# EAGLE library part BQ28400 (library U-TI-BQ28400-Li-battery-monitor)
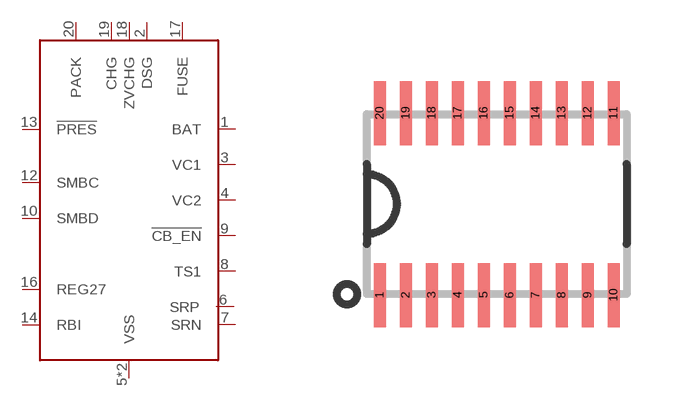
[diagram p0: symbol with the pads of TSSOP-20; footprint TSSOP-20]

Designator prefix U

## BQ28400  [TSSOP-20]
1  BAT  pwr
2  DSG  out
3  VC1  in
4  VC2  in
5  VSS  pwr
6  SRP  in
7  SRN  in
8  TS1  in
9  !CB_EN  out
10  SMBD
12  SMBC
13  !PRES  in
14  RBI  pwr
15  VSS  pwr
16  REG27  pwr
17  FUSE  out
18  ZVCHG  out
19  CHG  out
20  PACK  pwr

## Footprint TSSOP-20 (pad centres in mm)
smd 0.3 x 1.6: 1 -2.925,-2.275; 2 -2.275,-2.275; 3 -1.625,-2.275; 4 -0.975,-2.275; 5 -0.325,-2.275; 6 0.325,-2.275; 7 0.975,-2.275; 8 1.625,-2.275; 9 2.275,-2.275; 10 2.925,-2.275; 11 2.925,2.275; 12 2.275,2.275; 13 1.625,2.275; 14 0.975,2.275; 15 0.325,2.275; 16 -0.325,2.275; 17 -0.975,2.275; 18 -1.625,2.275; 19 -2.275,2.275; 20 -2.925,2.275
